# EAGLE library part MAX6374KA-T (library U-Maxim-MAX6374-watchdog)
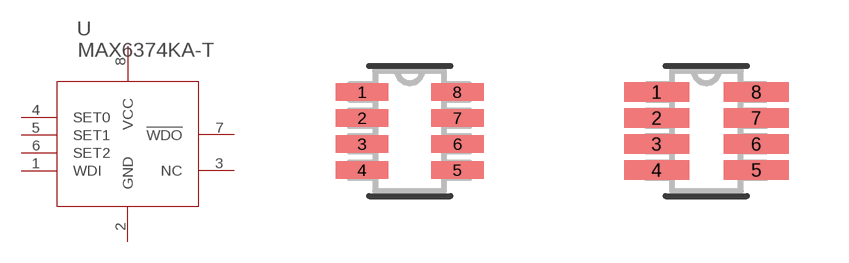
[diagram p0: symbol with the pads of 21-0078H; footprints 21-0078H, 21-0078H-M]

Designator prefix U

## MAX6374KA-T (MANUFACTURER_PART_NUMBER: max6374kat; VENDOR: Maxim Integrated Products)  [21-0078H]
1  WDI  in
2  GND  pwr
3  NC  nc
4  SET0  in
5  SET1  in
6  SET2  in
7  !WDO  out
8  VCC  pwr

## MAX6374KA-T21-0078H-M (MANUFACTURER_PART_NUMBER: max6374kat; VENDOR: Maxim Integrated Products)  [21-0078H-M]
Pads as for 21-0078H

## MAX6374KA-T21-0078H-L (MANUFACTURER_PART_NUMBER: max6374kat; VENDOR: Maxim Integrated Products)  [21-0078H-L]
Pads as for 21-0078H

## Footprint 21-0078H (pad centres in mm)
smd 1.321 x 0.432: 1 -1.194,0.975; 2 -1.194,0.325; 3 -1.194,-0.325; 4 -1.194,-0.975; 5 1.194,-0.975; 6 1.194,-0.325; 7 1.194,0.325; 8 1.194,0.975

## Footprint 21-0078H-M (pad centres in mm)
smd 1.626 x 0.483: 1 -1.245,0.975; 2 -1.245,0.325; 3 -1.245,-0.325; 4 -1.245,-0.975; 5 1.245,-0.975; 6 1.245,-0.325; 7 1.245,0.325; 8 1.245,0.975

## Footprint 21-0078H-L (pad centres in mm)
smd 1.016 x 0.381: 1 -1.143,0.975; 2 -1.143,0.325; 3 -1.143,-0.325; 4 -1.143,-0.975; 5 1.143,-0.975; 6 1.143,-0.325; 7 1.143,0.325; 8 1.143,0.975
